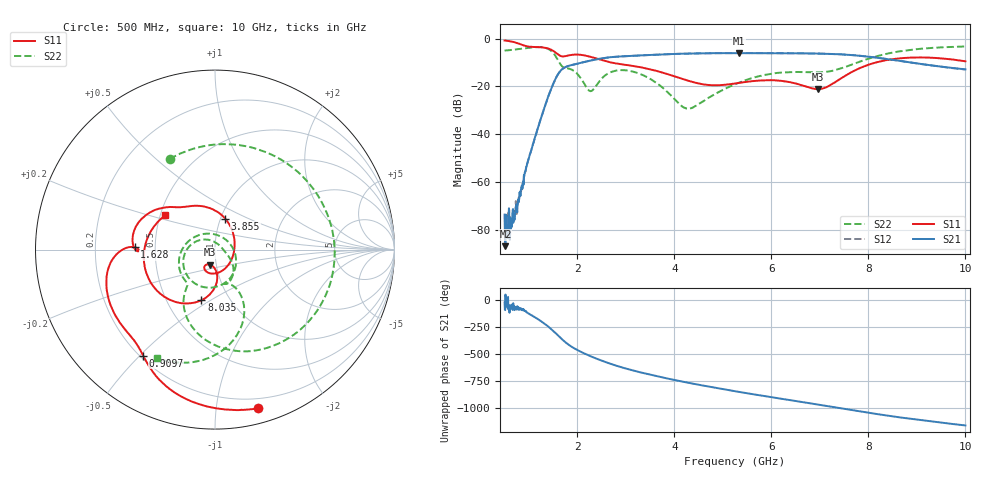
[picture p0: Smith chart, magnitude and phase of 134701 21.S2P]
!  2-Port S-parameters saved by WinCal
! VAR MeasName=S-Parameters (CALIBRATED_DATA) read from VNA (N5242A)
! VAR MeasDate=2013-7-3 16:31:29
! VAR NAME=134701 21
! VAR FILENAME=134701 21.S2P
! VAR DATE=2013-7-3 16:31:29
! VAR PHYS_PORTS=1,2
# Hz S MA R 50
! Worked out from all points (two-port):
!   1601 points, 500 MHz to 10 GHz, reference 50 ohm
!   highest |S21| = -6.02 dB at 5.339 GHz (marker M1); lowest = -86.8 dB at 517.8 MHz (marker M2)
!   |S21| within 3 dB of the highest: 2.302 GHz to 8.552 GHz (6.251 GHz wide, 115 % of centre)
!   lowest |S11| = -21.1 dB at 6.96 GHz (marker M3), VSWR 1.19, Z = 46.6 - j7.82 ohm
!   |S11| at or under -10 dB: 2.7 GHz to 8.15 GHz (5.451 GHz wide, 100 % of centre)
!   |S22| runs from -29.4 to -3.3 dB; largest |S21 - S12| = 0.0033
!   S11 on the Smith chart (normalised r, x): 500 MHz: 0.12, -1.30; 909.7 MHz: 0.21, -0.51; 1.628 GHz: 0.38, +0.01; 3.855 GHz: 1.05, +0.38; 8.035 GHz: 0.74, -0.46; 10 GHz: 0.53, +0.23
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5e8  0.9168 -74.8  0.0002086 -23.4  0.0001923 -56.6  0.5645 116.6
5.178125e8  0.9116 -77.3  4.549e-05 50.4  9.809e-05 -107.5  0.5663 114.1
6.721875e8  0.8572 -98.4  0.0002728 -72.8  0.0002051 -47.2  0.5843 91.3
9.096875e8  0.7135 -124.2  0.001402 -99.9  0.001468 -98.3  0.6253 50.5
1.165e9  0.6677 -143.1  0.01147 -171.8  0.01146 -172.1  0.6678 -4.0
1.372812e9  0.6312 -163.5  0.0515 123.3  0.05153 123.1  0.6263 -58.8
1.628125e9  0.4481 178.3  0.1981 18.7  0.1975 18.6  0.3162 -123.2
1.859688e9  0.4539 177.9  0.2774 -68.1  0.2767 -68.1  0.2302 -146.9
2.085312e9  0.4563 162.4  0.3145 -124.7  0.3138 -124.7  0.1412 153.5
2.287188e9  0.4124 149.1  0.3513 -165.5  0.3508 -165.5  0.08007 52.5
2.880938e9  0.2931 125.8  0.4238 98.5  0.423 98.4  0.2195 -111.1
3.670625e9  0.2065 84.3  0.4643 8.4  0.4635 8.4  0.111 154.5
3.854688e9  0.182 71.9  0.4725 -9.6  0.472 -9.5  0.07688 133.1
4.305938e9  0.1299 36.5  0.4879 -50.8  0.4881 -50.7  0.03428 43.1
5.25e9  0.1153 -53.5  0.4996 -127.7  0.5002 -127.8  0.1112 -34.9
5.339062e9  0.1191 -60.7  0.5 -134.5  0.5004 -134.6  0.1208 -37.8
6.0575e9  0.1346 -105.7  0.4964 172.8  0.4967 172.7  0.1885 -61.7
6.835312e9  0.09146 -116.6  0.4901 117.3  0.4903 117.3  0.1972 -74.1
6.96e9  0.08781 -108.7  0.4873 108.3  0.4881 108.2  0.1973 -72.5
8.034688e9  0.292 -105.0  0.4161 29.9  0.4167 29.7  0.3909 -65.3
8.420625e9  0.3617 -125.7  0.3698 3.6  0.3698 3.2  0.4929 -75.8
1e10  0.3361 145.2  0.2279 -85.9  0.2264 -86.2  0.686 -117.9
